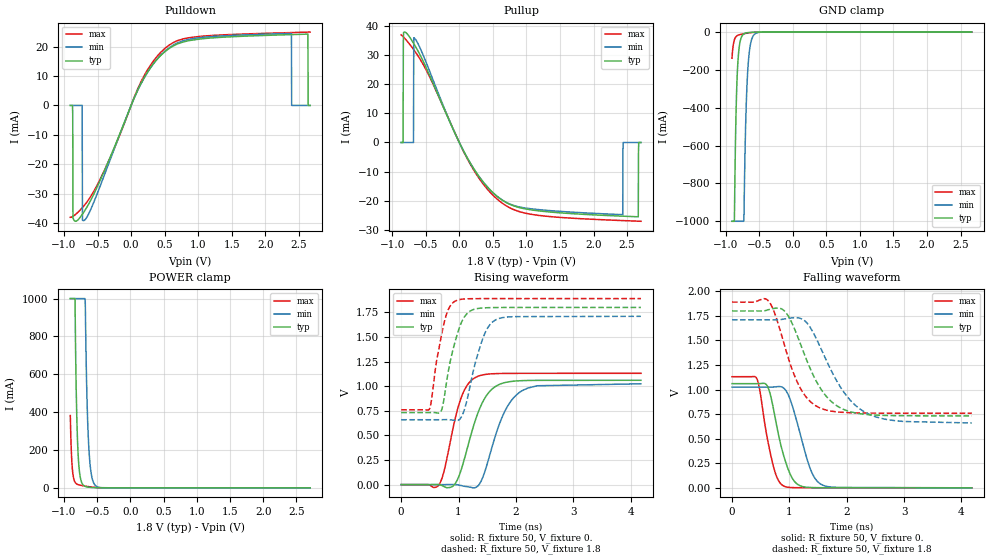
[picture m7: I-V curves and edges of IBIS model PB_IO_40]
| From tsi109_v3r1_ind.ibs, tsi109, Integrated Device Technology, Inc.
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|   MODEL PB_IO_40
[Model]   PB_IO_40
Model_type  I/O
Polarity   Non-Inverting
Enable   Active-High
|   typ   min   max
|C_comp_off 3.714p 3.449p 3.979p
|C_comp_on 4.164p 3.713p 4.513p
C_comp 3.939p 3.581p 4.246p
Vinl  =   0.300v
Vinh  =   1.500v
Vmeas =   0.9000V
Cref  =   1.0pF
Rref  =   50.0000
Vref  =   0.0V
[Model Spec]
[Temperature Range]   25   125   -40
[Voltage Range] 1.8 1.71 1.89
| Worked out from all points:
|   slope of the pulldown table from 0 to 0.27 V, typ, clamps not added: 22.1 ohm
|   slope of the pullup table from 0 to 0.27 V, typ, clamps not added: 24.6 ohm
|   GND clamp passes 1 mA (typ) near -0.59 V on its own axis
|   POWER clamp passes 1 mA (typ) near -0.54 V on its own axis
|   rising waveform, R_fixture 50, V_fixture 0.: 20-80 % time 351ps typ, 382ps min, 277ps max; typ from 0 V to 1.06 V
|   rising waveform, R_fixture 50, V_fixture 1.8: 20-80 % time 243ps typ, 281ps min, 201ps max; typ from 0.732 V to 1.8 V
|   falling waveform, R_fixture 50, V_fixture 0.: 20-80 % time 258ps typ, 298ps min, 210ps max; typ from 1.06 V to 0 V
|   falling waveform, R_fixture 50, V_fixture 1.8: 20-80 % time 512ps typ, 613ps min, 411ps max; typ from 1.8 V to 0.732 V
[Pulldown]
-906mV    0A         0A         -38.11mA
-866.3mV  -38.27mA   0A         -37.78mA
-826.6mV  -39.45mA   0A         -37.08mA
-729mV    -37.15mA   0A         -34.88mA
-725.4mV  -37.03mA   -39.06mA   -34.78mA
-696.5mV  -36.04mA   -39.11mA   -34.01mA
661.7mV   20.65mA    20.97mA    21.77mA
2.388V    24.12mA    24.53mA    24.8mA
2.392V    24.12mA    0A         24.81mA
2.634V    24.29mA    0A         24.97mA
2.638V    0A         0A         24.97mA
2.667V    0A         0A         24.99mA
[Pullup]
-866.6mV  0A         0A         37.11mA
-837.7mV  0A         0A         36.49mA
-834.1mV  34.47mA    0A         36.41mA
-816mV    38.07mA    0A         35.96mA
-682.3mV  34.23mA    0A         32.11mA
-675.1mV  33.95mA    36.08mA    31.87mA
740.9mV   -21.2mA    -21.1mA    -22.38mA
2.435V    -25.4mA    -24.88mA   -26.92mA
2.442V    -25.41mA   0A         -26.93mA
2.666V    -25.61mA   0A         -27.12mA
2.674V    0A         0A         -27.13mA
2.706V    0A         0A         -27.16mA
[GND Clamp]
-906mV    -1A        -1A        -138.5mA
-870.4mV  -1A        -1A        -41.43mA
-846.7mV  -443.6mA   -1A        -24.48mA
-818.9mV  -165.1mA   -1A        -17.07mA
-787.3mV  -54.66mA   -1A        -13.23mA
-731.8mV  -10.57mA   -1A        -8.987mA
-727.9mV  -9.631mA   -986.9mA   -8.726mA
-700.2mV  -5.362mA   -461.4mA   -6.989mA
-672.4mV  -3.349mA   -211.8mA   -5.424mA
-632.8mV  -1.859mA   -68.73mA   -3.516mA
-569.5mV  -686.7uA   -11.4mA    -1.394mA
2.667V    0A         0A         0A
[Power Clamp]
-906mV    1A         1A         382.4mA
-878.3mV  1A         1A         113.9mA
-835.1mV  996.9mA    1A         29.8mA
-816.6mV  504.7mA    1A         22.03mA
-791.9mV  201.6mA    1A         17.28mA
-758mV    59.94mA    1A         13.94mA
-702.4mV  11.79mA    1A         10.24mA
-680.9mV  7.51mA     979.8mA    8.974mA
-653.1mV  4.793mA    446.3mA    7.444mA
-622.2mV  3.19mA     184.3mA    5.874mA
-520.4mV  746.2uA    9.952mA    1.888mA
2.706V    0A         0A         0A
[Ramp]
dV/dt_r .636/350.688p .615/382.229p .679/277.286p
dV/dt_f .641/511.996p .631/613.561p .678/411.365p
[Rising Waveform]
R_fixture = 50
V_fixture = 0.
0s        0V         0V         0V
660ps     -377uV     -33.31uV   -835.1uV
970ps     37.1mV     -811.8uV   736.8mV
1.13ns    319.3mV    -18.86mV   989.8mV
1.31ns    682.1mV    -26.17mV   1.093V
1.43ns    848.8mV    84.6mV     1.116V
1.61ns    982.8mV    432.7mV    1.127V
1.83ns    1.04V      770.5mV    1.13V
2.09ns    1.056V     947.3mV    1.13V
4.18ns    1.06V      1.024V     1.131V
[Rising Waveform]
R_fixture = 50
V_fixture = 1.8
V_fixture_min = 1.71
V_fixture_max = 1.89
0s        731.7mV    659.2mV    759.6mV
500ps     731.9mV    659.2mV    777.1mV
710ps     764.9mV    659.6mV    1.538V
820ps     1.143V     660mV      1.775V
950ps     1.472V     651mV      1.867V
1.07ns    1.671V     710.7mV    1.885V
1.17ns    1.749V     913.8mV    1.888V
1.43ns    1.795V     1.495V     1.89V
1.65ns    1.799V     1.675V     1.89V
4.18ns    1.8V       1.71V      1.89V
[Falling Waveform]
R_fixture = 50
V_fixture = 0.
0s        1.06V      1.024V     1.131V
440ps     1.06V      1.024V     1.102V
640ps     1.005V     1.025V     432.1mV
770ps     660.6mV    1.029V     127.3mV
900ps     330.9mV    1.016V     19.31mV
1ns       158.6mV    920.8mV    4.531mV
1.12ns    46.82mV    698.4mV    1.475mV
1.36ns    3.689mV    201.6mV    384.1uV
1.56ns    1.25mV     33.8mV     130.8uV
4.18ns    0V         8.143uV    0V
[Falling Waveform]
R_fixture = 50
V_fixture = 1.8
V_fixture_min = 1.71
V_fixture_max = 1.89
0s        1.8V       1.71V      1.89V
620ps     1.81V      1.71V      1.911V
740ps     1.827V     1.709V     1.784V
900ps     1.807V     1.717V     1.482V
1.18ns    1.485V     1.726V     1.027V
1.34ns    1.246V     1.653V     892.5mV
1.52ns    1.034V     1.456V     816.8mV
1.94ns    799.9mV    982.5mV    767.9mV
2.36ns    746.1mV    756.9mV    760.9mV
4.18ns    731.7mV    660.1mV    759.6mV
